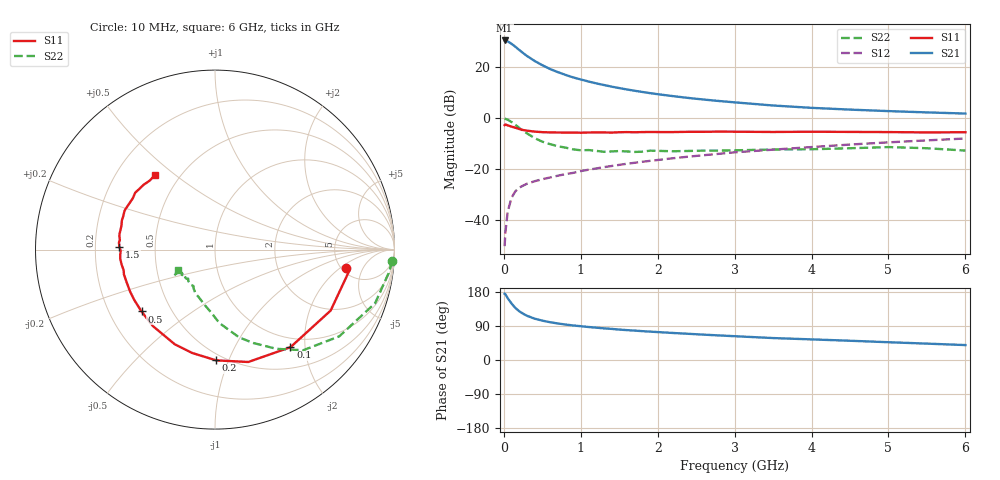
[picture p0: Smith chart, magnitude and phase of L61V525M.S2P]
!  INFINEON TECHNOLOGIES Small Signal Semiconductors
! BFR380L3 , Si-NPN RF-Transistor in TSLP-3-1
!  Vce=1.5 V,  Ic=25 mA
! Common Emitter S-Parameters:  07. March 2005
#  GHz  S  MA  R  50
! f  S11  S21  S12  S22
! GHz  Mag  Ang  Mag  Ang  Mag  Ang  Mag  Ang
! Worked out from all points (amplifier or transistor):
!   36 points, 10 MHz to 6 GHz, reference 50 ohm
!   highest |S21| = 30.6 dB at 10 MHz (marker M1)
!   |S21| within 3 dB of that: start of sweep to 171.2 MHz
!   unconditionally stable (mu >= 1): 1.886 GHz to 4.931 GHz
!   at 250 MHz: K = 0.38, MSG = 26.0 dB, |S12| = -26.4 dB
!   at 1.4 GHz: K = 0.96, MSG = 15.6 dB, |S12| = -18.7 dB
!   at 6 GHz: K = 0.98, MSG = 4.9 dB, |S12| = -7.9 dB
!   S11 on the Smith chart (normalised r, x): 10 MHz: 5.41, -2.43; 100 MHz: 0.84, -1.72; 200 MHz: 0.45, -0.90; 500 MHz: 0.34, -0.33; 1.5 GHz: 0.30, +0.01; 6 GHz: 0.37, +0.43
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0.01  0.7345 -8.1  33.73 174.8  0.0031 84.0  0.9896 -3.7
0.02  0.7584 -8.7  33.52 173.4  0.0057 87.0  0.9763 -7.7
0.05  0.7284 -27.8  32.34 163.3  0.0147 78.2  0.9407 -18.5
0.1  0.6873 -52.3  29.01 149.0  0.0277 68.4  0.8445 -34.9
0.15  0.6531 -73.5  25.4 137.4  0.037 60.1  0.7454 -48.8
0.2  0.6172 -89.4  21.96 128.7  0.0436 55.9  0.6496 -58.3
0.25  0.5898 -102.4  19.16 122.2  0.0478 52.3  0.5632 -67.6
0.3  0.5732 -113.0  16.76 116.8  0.052 50.7  0.5076 -74.6
0.4  0.5489 -129.1  13.37 109.1  0.0583 49.2  0.4098 -86.6
0.5  0.5353 -139.9  11.03 103.9  0.0638 50.4  0.3483 -93.9
0.6  0.5302 -148.1  9.303 99.7  0.069 51.4  0.3118 -101.1
0.8  0.5248 -159.9  7.136 93.6  0.0803 53.8  0.2664 -114.2
0.9  0.5259 -164.8  6.361 91.2  0.085 55.6  0.2468 -118.9
1.1  0.5271 -171.0  5.278 87.1  0.0981 57.5  0.2385 -125.0
1.5  0.5333 178.2  3.924 80.3  0.1221 60.2  0.228 -135.2
1.8  0.5373 172.2  3.294 76.1  0.1404 61.2  0.2216 -140.6
2.2  0.5378 165.8  2.724 71.3  0.1648 62.0  0.2259 -143.4
2.8  0.5486 156.8  2.185 64.8  0.2014 62.3  0.2325 -149.3
3.5  0.5397 148.1  1.785 57.9  0.2428 60.8  0.2441 -148.5
4.5  0.5411 141.7  1.483 50.8  0.3058 59.4  0.2588 -148.0
5.5  0.5292 133.4  1.307 43.2  0.3692 55.8  0.2589 -148.2
6  0.5338 128.4  1.241 39.4  0.4021 53.8  0.2328 -151.5
